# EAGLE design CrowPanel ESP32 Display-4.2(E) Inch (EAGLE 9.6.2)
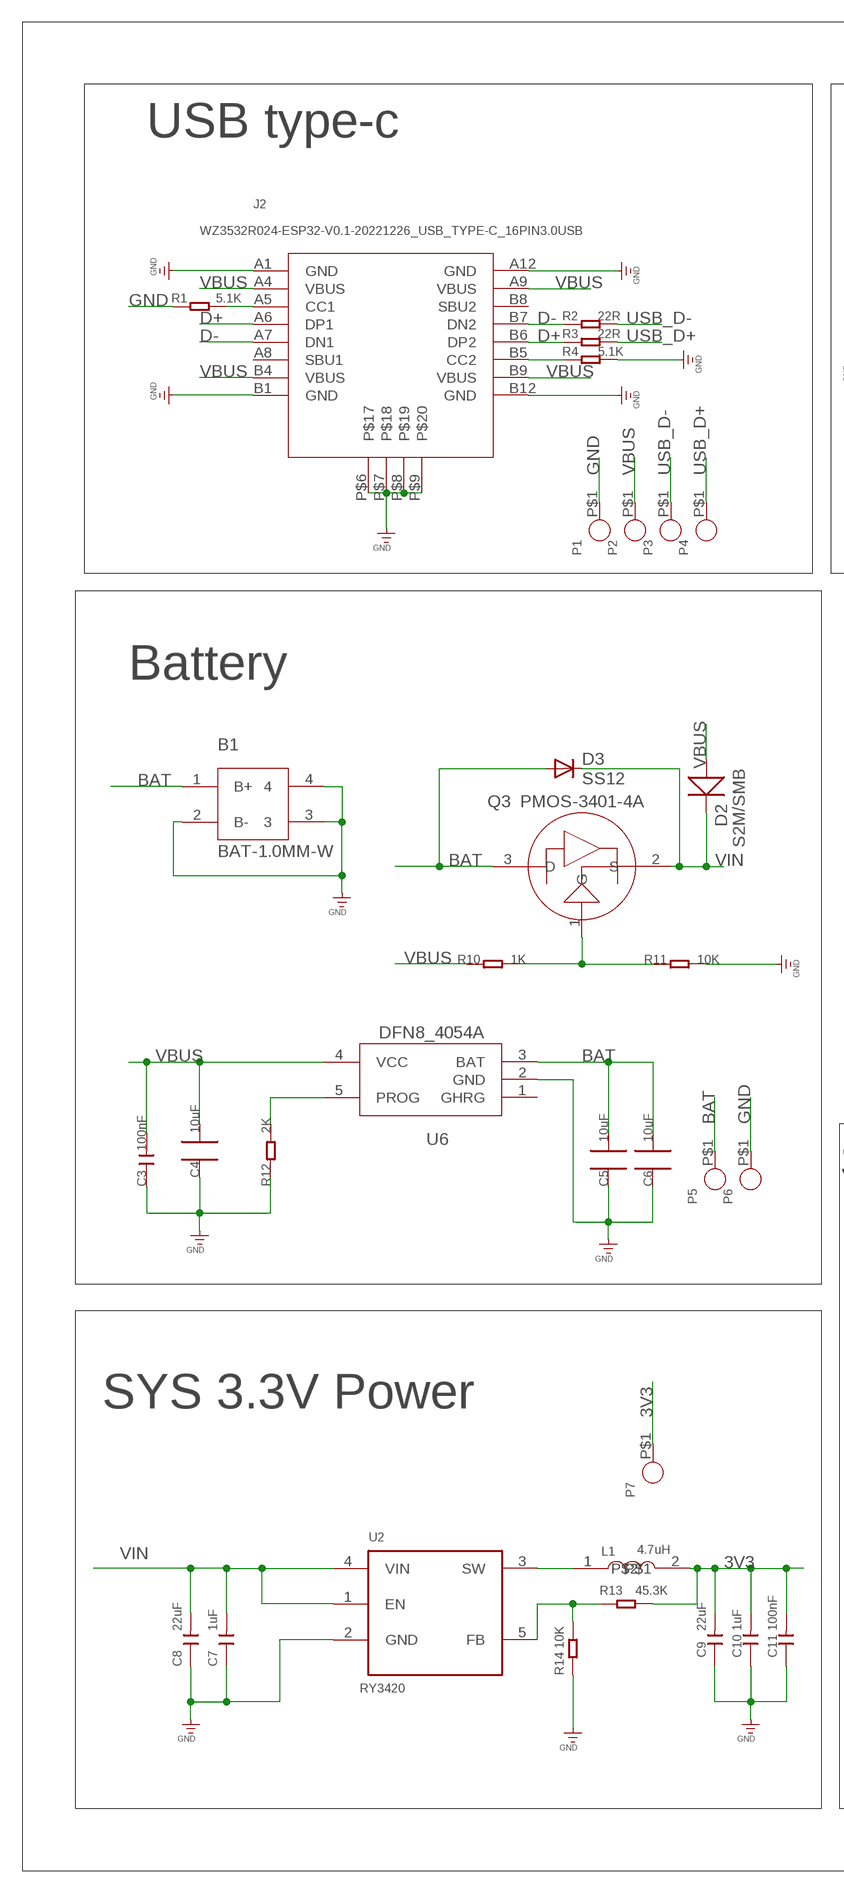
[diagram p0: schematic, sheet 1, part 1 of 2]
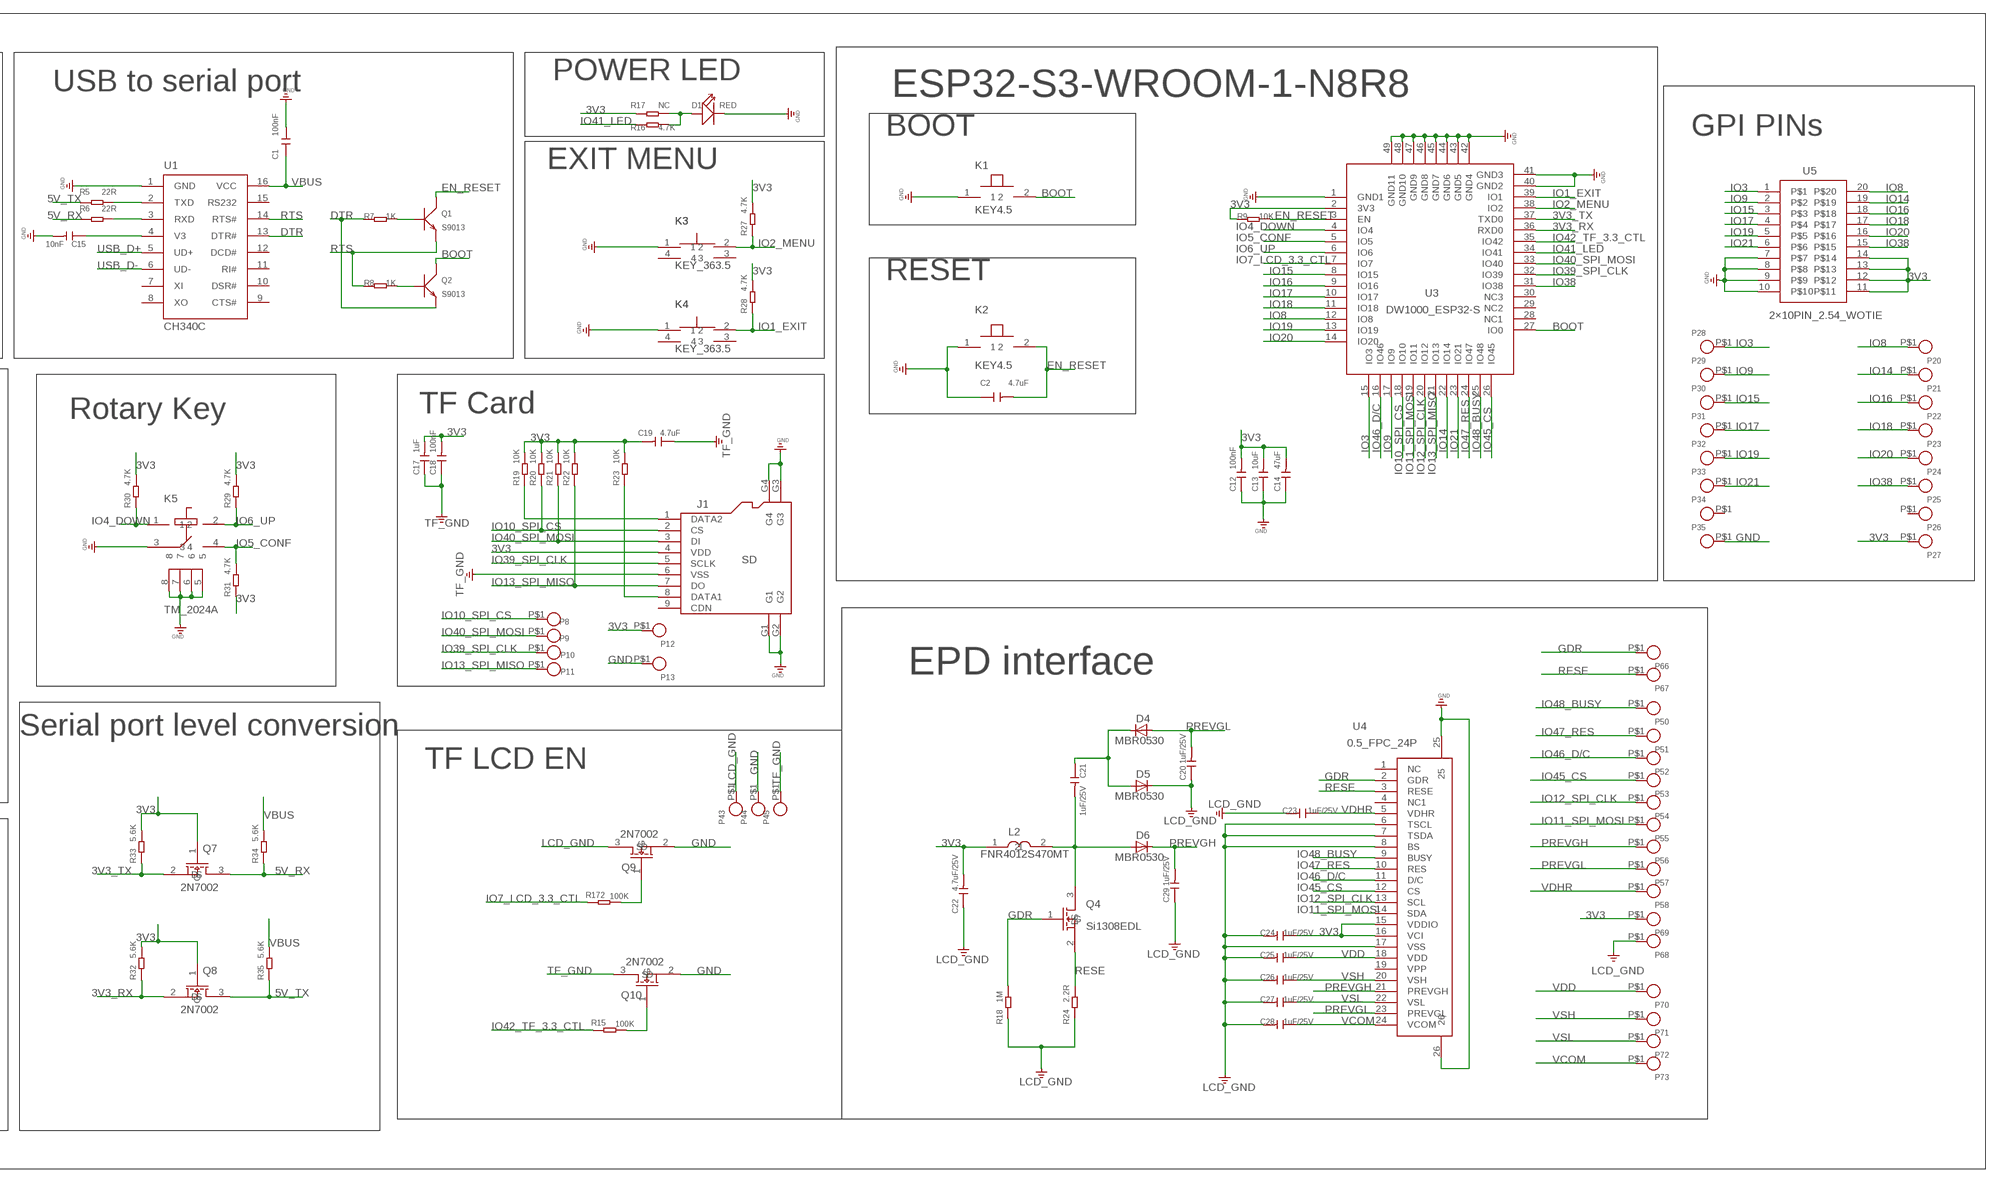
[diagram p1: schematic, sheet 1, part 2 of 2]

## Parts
B1  BAT-1.0MM-W  [SH1.0MM-W]
C1  100nF  C0603  [0603]
C2  4.7uF  A_XBJ_C0603  [A_XBJ_0603]
C3  100nF  A9G_DISCRETE_C-0603  [A9G_DISCRETE_C0603]
C4  10uF  CPT_SMD_C0805_S  [CPT_SMD_0805_S]
C5  10uF  CPT_SMD_C0805_S  [CPT_SMD_0805_S]
C6  10uF  CPT_SMD_C0805_S  [CPT_SMD_0805_S]
C7  1uF  A_XBJ_C0603  [A_XBJ_0603]
C8  22uF  A_XBJ_C0805  [A_XBJ_0805]
C9  22uF  A_XBJ_C0805  [A_XBJ_0805]
C10  1uF  A_XBJ_C0603  [A_XBJ_0603]
C11  100nF  A_XBJ_C0603  [A_XBJ_0603]
C12  100nF  A9G_DISCRETE_C-0603  [A9G_DISCRETE_C0603]
C13  10uF  A9G_DISCRETE_C-0603  [A9G_DISCRETE_C0603]
C14  47uF  A9G_DISCRETE_C-0805  [A9G_DISCRETE_C0805]
C15  10nF  A_XBJ_C0603  [A_XBJ_0603]
C17  1uF  A9G_DISCRETE_C-0603  [A9G_DISCRETE_C0603]
C18  100nF  A9G_DISCRETE_C-0603  [A9G_DISCRETE_C0603]
C19  4.7uF  A9G_DISCRETE_C-0603  [A9G_DISCRETE_C0603]
C20  1uF/25V  A9G_DISCRETE_C-0603  [A9G_DISCRETE_C0603]
C21  1uF/25V  A9G_DISCRETE_C-0603  [A9G_DISCRETE_C0603]
C22  4.7uF/25V  A9G_DISCRETE_C-0603  [A9G_DISCRETE_C0603]
C23  1uF/25V  A9G_DISCRETE_C-0603  [A9G_DISCRETE_C0603]
C24  1uF/25V  A9G_DISCRETE_C-0603  [A9G_DISCRETE_C0603]
C25  1uF/25V  A9G_DISCRETE_C-0603  [A9G_DISCRETE_C0603]
C26  1uF/25V  A9G_DISCRETE_C-0603  [A9G_DISCRETE_C0603]
C27  1uF/25V  A9G_DISCRETE_C-0603  [A9G_DISCRETE_C0603]
C28  1uF/25V  A9G_DISCRETE_C-0603  [A9G_DISCRETE_C0603]
C29  1uF/25V  A9G_DISCRETE_C-0603  [A9G_DISCRETE_C0603]
D1  RED  A_XBJ_DISCRETE_LED0603  [A_XBJ_DISCRETE_LED-0603]
D2  S2M/SMB  DO-214AB_214ABDO-214AB  [DO-214AB_214AB]
D3  SS12  DIODE_DIODE-DO-214AC  [DIODE_DO-214AC]
D4  MBR0530  DIODE_DIODE-SOD123  [DIODE_SOD123]
D5  MBR0530  DIODE_DIODE-SOD123  [DIODE_SOD123]
D6  MBR0530  DIODE_DIODE-SOD123  [DIODE_SOD123]
J1  SD  CONNECTOR_HOLDER-MICROSD-9P  [CONNECTOR_9P-SMD-W/-RING]
J2  WZ3532R024-ESP32-V0.1-20221226_USB_TYPE-C_16PIN3.0USB  [WZ3532R024-ESP32-V0.1-20221226_KEVIN_3.0TYPEC-SMD]
K1  KEY4.5  [KEY-4.5]
K2  KEY4.5  [KEY-4.5]
K3  KEY_363.5  [KEY_3*6*3.5]
K4  KEY_363.5  [KEY_3*6*3.5]
K5  TM_2024A  [TM_2024A]
L1  4.7uH  WZ2432R028-ESP32-V1.2-20231108_L-0530  [WZ2432R028-ESP32-V1.2-20231108_CD54_CD54]
L2  FNR4012S470MT  [FNR4012S470MT]
P1  CROWPI_POW_PADPAD-1.0MM  [CROWPI_POW_PAD-1.0MM]
P2  CROWPI_POW_PADPAD-1.0MM  [CROWPI_POW_PAD-1.0MM]
P3  CROWPI_POW_PADPAD-1.0MM  [CROWPI_POW_PAD-1.0MM]
P4  CROWPI_POW_PADPAD-1.0MM  [CROWPI_POW_PAD-1.0MM]
P5  CROWPI_POW_PADPAD-1.0MM  [CROWPI_POW_PAD-1.0MM]
P6  CROWPI_POW_PADPAD-1.0MM  [CROWPI_POW_PAD-1.0MM]
P7  CROWPI_POW_PADPAD-1.0MM  [CROWPI_POW_PAD-1.0MM]
P8  CROWPI_POW_PADPAD-1.0MM  [CROWPI_POW_PAD-1.0MM]
P9  CROWPI_POW_PADPAD-1.0MM  [CROWPI_POW_PAD-1.0MM]
P10  CROWPI_POW_PADPAD-1.0MM  [CROWPI_POW_PAD-1.0MM]
P11  CROWPI_POW_PADPAD-1.0MM  [CROWPI_POW_PAD-1.0MM]
P12  CROWPI_POW_PADPAD-1.0MM  [CROWPI_POW_PAD-1.0MM]
P13  CROWPI_POW_PADPAD-1.0MM  [CROWPI_POW_PAD-1.0MM]
P20  CROWPI_POW_PADPAD-1.0MM  [CROWPI_POW_PAD-1.0MM]
P21  CROWPI_POW_PADPAD-1.0MM  [CROWPI_POW_PAD-1.0MM]
P22  CROWPI_POW_PADPAD-1.0MM  [CROWPI_POW_PAD-1.0MM]
P23  CROWPI_POW_PADPAD-1.0MM  [CROWPI_POW_PAD-1.0MM]
P24  CROWPI_POW_PADPAD-1.0MM  [CROWPI_POW_PAD-1.0MM]
P25  CROWPI_POW_PADPAD-1.0MM  [CROWPI_POW_PAD-1.0MM]
P26  CROWPI_POW_PADPAD-1.0MM  [CROWPI_POW_PAD-1.0MM]
P27  CROWPI_POW_PADPAD-1.0MM  [CROWPI_POW_PAD-1.0MM]
P28  CROWPI_POW_PADPAD-1.0MM  [CROWPI_POW_PAD-1.0MM]
P29  CROWPI_POW_PADPAD-1.0MM  [CROWPI_POW_PAD-1.0MM]
P30  CROWPI_POW_PADPAD-1.0MM  [CROWPI_POW_PAD-1.0MM]
P31  CROWPI_POW_PADPAD-1.0MM  [CROWPI_POW_PAD-1.0MM]
P32  CROWPI_POW_PADPAD-1.0MM  [CROWPI_POW_PAD-1.0MM]
P33  CROWPI_POW_PADPAD-1.0MM  [CROWPI_POW_PAD-1.0MM]
P34  CROWPI_POW_PADPAD-1.0MM  [CROWPI_POW_PAD-1.0MM]
P35  CROWPI_POW_PADPAD-1.0MM  [CROWPI_POW_PAD-1.0MM]
P43  CROWPI_POW_PADPAD-1.0MM  [CROWPI_POW_PAD-1.0MM]
P44  CROWPI_POW_PADPAD-1.0MM  [CROWPI_POW_PAD-1.0MM]
P45  CROWPI_POW_PADPAD-1.0MM  [CROWPI_POW_PAD-1.0MM]
P50  CROWPI_POW_PADPAD-1.0MM  [CROWPI_POW_PAD-1.0MM]
P51  CROWPI_POW_PADPAD-1.0MM  [CROWPI_POW_PAD-1.0MM]
P52  CROWPI_POW_PADPAD-1.0MM  [CROWPI_POW_PAD-1.0MM]
P53  CROWPI_POW_PADPAD-1.0MM  [CROWPI_POW_PAD-1.0MM]
P54  CROWPI_POW_PADPAD-1.0MM  [CROWPI_POW_PAD-1.0MM]
P55  CROWPI_POW_PADPAD-1.0MM  [CROWPI_POW_PAD-1.0MM]
P56  CROWPI_POW_PADPAD-1.0MM  [CROWPI_POW_PAD-1.0MM]
P57  CROWPI_POW_PADPAD-1.0MM  [CROWPI_POW_PAD-1.0MM]
P58  CROWPI_POW_PADPAD-1.0MM  [CROWPI_POW_PAD-1.0MM]
P66  CROWPI_POW_PADPAD-1.0MM  [CROWPI_POW_PAD-1.0MM]
P67  CROWPI_POW_PADPAD-1.0MM  [CROWPI_POW_PAD-1.0MM]
P68  CROWPI_POW_PADPAD-1.0MM  [CROWPI_POW_PAD-1.0MM]
P69  CROWPI_POW_PADPAD-1.0MM  [CROWPI_POW_PAD-1.0MM]
P70  CROWPI_POW_PADPAD-1.0MM  [CROWPI_POW_PAD-1.0MM]
P71  CROWPI_POW_PADPAD-1.0MM  [CROWPI_POW_PAD-1.0MM]
P72  CROWPI_POW_PADPAD-1.0MM  [CROWPI_POW_PAD-1.0MM]
P73  CROWPI_POW_PADPAD-1.0MM  [CROWPI_POW_PAD-1.0MM]
Q1  S9013  DISCRETE_TRANSISTOR-NPN-SOT23  [DISCRETE_SOT23$1]
Q2  S9013  DISCRETE_TRANSISTOR-NPN-SOT23  [DISCRETE_SOT23$1]
Q3  PMOS-3401-4A  DFN8_P-MOS-SOT23  [DFN8_SOT-23]
Q4  Si1308EDL  HXY2102EI  [SOT-323_W]
Q7  2N7002  NMOS_W  [SOT23-3_W]
Q8  2N7002  NMOS_W  [SOT23-3_W]
Q9  2N7002  NMOS_W  [SOT23-3_W]
Q10  2N7002  NMOS_W  [SOT23-3_W]
R1  5.1K  R0603  [R0603]
R2  22R  R0603  [R0603]
R3  22R  R0603  [R0603]
R4  5.1K  R0603  [R0603]
R5  22R  R0603  [R0603]
R6  22R  R0603  [R0603]
R7  1K  A9G_DISCRETE_R-0603  [A9G_DISCRETE_R0603]
R8  1K  A9G_DISCRETE_R-0603  [A9G_DISCRETE_R0603]
R9  10K  A9G_DISCRETE_R-0603  [A9G_DISCRETE_R0603]
R10  1K  A9G_DISCRETE_R-0603  [A9G_DISCRETE_R0603]
R11  10K  A9G_DISCRETE_R-0603  [A9G_DISCRETE_R0603]
R12  2K  A9G_DISCRETE_R-0603  [A9G_DISCRETE_R0603]
R13  45.3K  A9G_DISCRETE_R-0603  [A9G_DISCRETE_R0603]
R14  10K  A9G_DISCRETE_R-0603  [A9G_DISCRETE_R0603]
R15  100K  R-0603  [R0603]
R16  4.7K  A9G_DISCRETE_R-0603  [A9G_DISCRETE_R0603]
R17  NC  A9G_DISCRETE_R-0603  [A9G_DISCRETE_R0603]
R18  1M  A9G_DISCRETE_R-0603  [A9G_DISCRETE_R0603]
R19  10K  A9G_DISCRETE_R-0603  [A9G_DISCRETE_R0603]
R20  10K  A9G_DISCRETE_R-0603  [A9G_DISCRETE_R0603]
R21  10K  A9G_DISCRETE_R-0603  [A9G_DISCRETE_R0603]
R22  10K  A9G_DISCRETE_R-0603  [A9G_DISCRETE_R0603]
R23  10K  A9G_DISCRETE_R-0603  [A9G_DISCRETE_R0603]
R24  2.2R  A9G_DISCRETE_R-0603  [A9G_DISCRETE_R0603]
R27  4.7K  A9G_DISCRETE_R-0603  [A9G_DISCRETE_R0603]
R28  4.7K  A9G_DISCRETE_R-0603  [A9G_DISCRETE_R0603]
R29  4.7K  A9G_DISCRETE_R-0603  [A9G_DISCRETE_R0603]
R30  4.7K  A9G_DISCRETE_R-0603  [A9G_DISCRETE_R0603]
R31  4.7K  A9G_DISCRETE_R-0603  [A9G_DISCRETE_R0603]
R32  5.6K  DISCRETE_R-0603  [DISCRETE_R0603]
R33  5.6K  DISCRETE_R-0603  [DISCRETE_R0603]
R34  5.6K  DISCRETE_R-0603  [DISCRETE_R0603]
R35  5.6K  DISCRETE_R-0603  [DISCRETE_R0603]
R172  100K  R-0603  [R0603]
U1  CH340C  A_XBJ_CH340G  [A_XBJ_SOP-16]
U2  RY3420  CROWBOT_-V1.0-20220525_A_XBJ_HM3420B  [CROWBOT_-V1.0-20220525_A_XBJ_SOT23-5]
U3  DW1000_ESP32-S  [DW1000_ESP32-S3]
U4  0.5_FPC_24P  [0.5_FPC_24P]
U5  2×10PIN_2.54_WOTIE  [2*10PIN_2.54_WOTIE]
U6  DFN8_4054A  [DFN8_SOP23-5]

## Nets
3V3: C9.2 C10.2 C11.2 C12.2 C13.2 C14.2 C17.2 C18.2 C19.2 C22.2 C24.1 J1.4(VDD) L1.2 L2.1 P7.P$1 P12.P$1 P27.P$1 P69.P$1 Q7.1(G) Q8.1(G) R9.1 R13.2 R17.1 R19.2 R20.2 R21.2 R22.2 R23.2 R27.2 R28.2 R29.2 R30.2 R31.1 R32.2 R33.2 U3.2(3V3) U4.15(VDDIO) U4.16(VCI) U5.11 U5.12 U5.13 U5.14
3V3_RX: Q8.2(S) R32.1 U3.36(RXD0)
3V3_TX: Q7.2(S) R33.1 U3.37(TXD0)
5V_RX: Q7.3(D) R6.1 R34.1
5V_TX: Q8.3(D) R5.1 R35.1
BAT: B1.1(B+) C5.2 C6.2 D3.A P5.P$1 Q3.3(D) U6.3(BAT)
BOOT: K1.2 Q2.3(C) U3.27(IO0)
D+: J2.A6(DP1) J2.B6(DP2) R3.1
D-: J2.A7(DN1) J2.B7(DN2) R2.1
DTR: Q2.2(E) R7.1 U1.13(DTR#)
EN_RESET: C2.2 K2.2 Q1.3(C) R9.2 U3.3(EN)
GDR: P66.P$1 Q4.1(G) R18.2 U4.2(GDR)
GND: B1.2(B-) B1.3 B1.4 C1.2 C2.1 C3.1 C4.1 C5.1 C6.1 C7.1 C8.1 C9.1 C10.1 C11.1 C12.1 C13.1 C14.1 C15.2 D1.- J1.G1 J1.G2 J1.G3 J1.G4 J2.A1(GND) J2.A12(GND) J2.B1(GND) J2.B12(GND) J2.P$6 J2.P$7 J2.P$8 J2.P$9 K1.1 K2.1 K3.1 K4.1 K5.3 K5.5 K5.6 K5.7 K5.8 P1.P$1 P6.P$1 P13.P$1 P35.P$1 P44.P$1 Q9.2(S) Q10.2(S) R1.1 R4.2 R11.2 R12.1 R14.1 U1.1(GND) U2.2(GND) U3.1(GND1) U3.40(GND2) U3.41(GND3) U3.42(GND4) U3.43(GND5) U3.44(GND6) U3.45(GND7) U3.46(GND8) U3.47(GND9) U3.48(GND10) U3.49(GND11) U4.25 U4.26 U5.7 U5.8 U5.9 U5.10 U6.2(GND)
IO1_EXIT: K4.2 R28.1 U3.39(IO1)
IO2_MENU: K3.2 R27.1 U3.38(IO2)
IO3: P28.P$1 U3.15(IO3) U5.1
IO4_DOWN: K5.1 R30.1 U3.4(IO4)
IO5_CONF: K5.4 R31.2 U3.5(IO5)
IO6_UP: K5.2 R29.1 U3.6(IO6)
IO7_LCD_3.3_CTL: R172.1 U3.7(IO7)
IO8: P20.P$1 U3.12(IO8) U5.20
IO9: P29.P$1 U3.17(IO9) U5.2
IO10_SPI_CS: J1.2(CS) P8.P$1 R20.1 U3.18(IO10)
IO11_SPI_MOSI: P55.P$1 U3.19(IO11) U4.14(SDA)
IO12_SPI_CLK: P54.P$1 U3.20(IO12) U4.13(SCL)
IO13_SPI_MISO: J1.7(DO) P11.P$1 R22.1 U3.21(IO13)
IO14: P21.P$1 U3.22(IO14) U5.19
IO15: P30.P$1 U3.8(IO15) U5.3
IO16: P22.P$1 U3.9(IO16) U5.18
IO17: P31.P$1 U3.10(IO17) U5.4
IO18: P23.P$1 U3.11(IO18) U5.17
IO19: P32.P$1 U3.13(IO19) U5.5
IO20: P24.P$1 U3.14(IO20) U5.16
IO21: P33.P$1 U3.23(IO21) U5.6
IO38: P25.P$1 U3.31(IO38) U5.15
IO39_SPI_CLK: J1.5(SCLK) P10.P$1 U3.32(IO39)
IO40_SPI_MOSI: J1.3(DI) P9.P$1 R21.1 U3.33(IO40)
IO41_LED: R16.1 U3.34(IO41)
IO42_TF_3.3_CTL: R15.1 U3.35(IO42)
IO45_CS: P53.P$1 U3.26(IO45) U4.12(CS)
IO46_D/C: P52.P$1 U3.16(IO46) U4.11(D/C)
IO47_RES: P51.P$1 U3.24(IO47) U4.10(RES)
IO48_BUSY: P50.P$1 U3.25(IO48) U4.9(BUSY)
LCD_GND: C20.1 C22.1 C23.2 C24.2 C25.2 C26.2 C27.2 C28.2 C29.1 D5.C P43.P$1 P68.P$1 Q9.3(D) R18.1 R24.1 U4.6(TSCL) U4.7(TSDA) U4.8(BS) U4.17(VSS) ; supply symbol labelled GND
N$1: Q1.1(B) R7.2
N$2: R5.2 U1.2(TXD)
N$3: R6.2 U1.3(RXD)
N$4: Q2.1(B) R8.2
N$5: J2.A5(CC1) R1.2
N$6: Q3.1(G) R10.2 R11.1
N$7: Q9.1(G) R172.2
N$8: Q10.1(G) R15.2
N$9: R13.1 R14.2 U2.5(FB)
N$10: J1.1(DATA2) R19.1
N$11: L1.1 U2.3(SW)
N$12: J2.B5(CC2) R4.1
N$13: C15.1 U1.4(V3)
N$16: R12.2 U6.5(PROG)
N$20: J1.8(DATA1) R23.1
N$25: D1.+ R16.2 R17.2
N$55: C21.1 D4.C D5.A
N$56: C21.2 D6.A L2.2 Q4.3(D)
PREVGH: C29.2 D6.C P56.P$1 U4.21(PREVGH)
PREVGL: C20.2 D4.A P57.P$1 U4.23(PREVGL)
RESE: P67.P$1 Q4.2(S) R24.2 U4.3(RESE)
RTS: Q1.2(E) R8.1 U1.14(RTS#)
TF_GND: C17.1 C18.1 C19.1 J1.6(VSS) P45.P$1 Q10.3(D) ; supply symbol labelled GND
USB_D+: P4.P$1 R3.2 U1.5(UD+)
USB_D-: P3.P$1 R2.2 U1.6(UD-)
VBUS: C1.1 C3.2 C4.2 D2.1(+) J2.A4(VBUS) J2.A9(VBUS) J2.B4(VBUS) J2.B9(VBUS) P2.P$1 R10.1 R34.2 R35.2 U1.16(VCC) U6.4(VCC)
VCOM: C28.1 P73.P$1 U4.24(VCOM)
VDD: C25.1 P70.P$1 U4.18(VDD)
VDHR: C23.1 P58.P$1 U4.5(VDHR)
VIN: C7.2 C8.2 D2.2(-) D3.C Q3.2(S) U2.1(EN) U2.4(VIN)
VSH: C26.1 P71.P$1 U4.20(VSH)
VSL: C27.1 P72.P$1 U4.22(VSL)
Unconnected: J1.9(CDN) J2.A8(SBU1) J2.B8(SBU2) K3.3 K3.4 K4.3 K4.4 P26.P$1 P34.P$1 U1.7(XI) U1.8(XO) U1.9(CTS#) U1.10(DSR#) U1.11(RI#) U1.12(DCD#) U1.15(RS232) U3.28(NC1) U3.29(NC2) U3.30(NC3) U4.1(NC) U4.4(NC1) U4.19(VPP) U6.1(GHRG)

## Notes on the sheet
- USB type-c | POWER LED
- USB to serial port | ESP32-S3-WROOM-1-N8R8
- BOOT | GPI PINs
- EXIT MENU
- RESET
- Rotary Key | TF Card
- Battery
- EPD interface
- Serial port level conversion
- TF LCD EN
- SYS 3.3V Power

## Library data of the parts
B1 = WGH:BAT-1.0MM-W
C1 = WGH:C0603
C2 C7 C10 C11 C15 = CrowPanel ESP32 Display-4.3-inch-V2.1-20240314:A_XBJ_C0603
C3 C12-C14 C17-C29 = CrowPanel ESP32 Display-4.3-inch-V2.1-20240314:A9G_DISCRETE_C*: Ceramic Capacitors
C4-C6 = CrowPanel ESP32 Display-4.3-inch-V2.1-20240314:CPT_SMD_C0805
C8 C9 = CrowPanel ESP32 Display-4.3-inch-V2.1-20240314:A_XBJ_C0805
D1 = CrowPanel ESP32 Display-4.3-inch-V2.1-20240314:A_XBJ_DISCRETE_LED*
D2 = CrowPanel ESP32 Display-4.3-inch-V2.1-20240314:DO-214AB_214AB: 214AB
D3-D6 = CrowPanel ESP32 Display-4.3-inch-V2.1-20240314:DIODE_DIODE-: DIODE
J1 = CrowPanel ESP32 Display-4.3-inch-V2.1-20240314:CONNECTOR_HOLDER-MICROSD-9P
J2 = CrowPanel ESP32 Display-4.3-inch-V2.1-20240314:WZ3532R024-ESP32-V0.1-20221226_USB_TYPE-C_16PIN
K1 K2 = WGH:KEY4.5
K3 K4 = WGH:KEY_3*6*3.5
K5 = WGH:TM_2024A
L1 = CrowPanel ESP32 Display-4.3-inch-V2.1-20240314:WZ2432R028-ESP32-V1.2-20231108_L-0530
L2 = WGH:FNR4012S470MT
P1-P13 P20-P35 P43-P45 P50-P58 P66-P73 = ESP32 Terminal - 3.5 Inch_2.0:CROWPI_POW_PAD*
Q1 Q2 = CrowPanel ESP32 Display-4.3-inch-V2.1-20240314:DISCRETE_TRANSISTOR-NPN*: NPN audion
Q3 = CrowPanel ESP32 Display-4.3-inch-V2.1-20240314:DFN8_P-MOS-SOT23
Q4 = WGH:HXY2102EI
Q7-Q10 = WGH:NMOS_W
R1-R6 = WGH:R0603
R7-R14 R16-R24 R27-R31 = CrowPanel ESP32 Display-4.3-inch-V2.1-20240314:A9G_DISCRETE_R*
R15 R172 = discrete:R*
R32-R35 = CrowPanel ESP32 Display-4.3-inch-V2.1-20240314:DISCRETE_R*
U1 = CrowPanel ESP32 Display-4.3-inch-V2.1-20240314:A_XBJ_CH340G
U2 = CrowPanel ESP32 Display-4.3-inch-V2.1-20240314:CROWBOT_-V1.0-20220525_A_XBJ_HM3420B
U3 = CrowPanel ESP32 Display-4.3-inch-V2.1-20240314:DW1000_ESP32-S
U4 = ESP32 Terminal - 3.5 Inch_2.0:0.5_FPC_24P
U5 = WGH:2×10PIN_2.54_WOTIE
U6 = CrowPanel ESP32 Display-4.3-inch-V2.1-20240314:DFN8_4054A

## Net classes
0 default: width 0.254 mm, drill 0.305 mm, clearance 0.152 mm

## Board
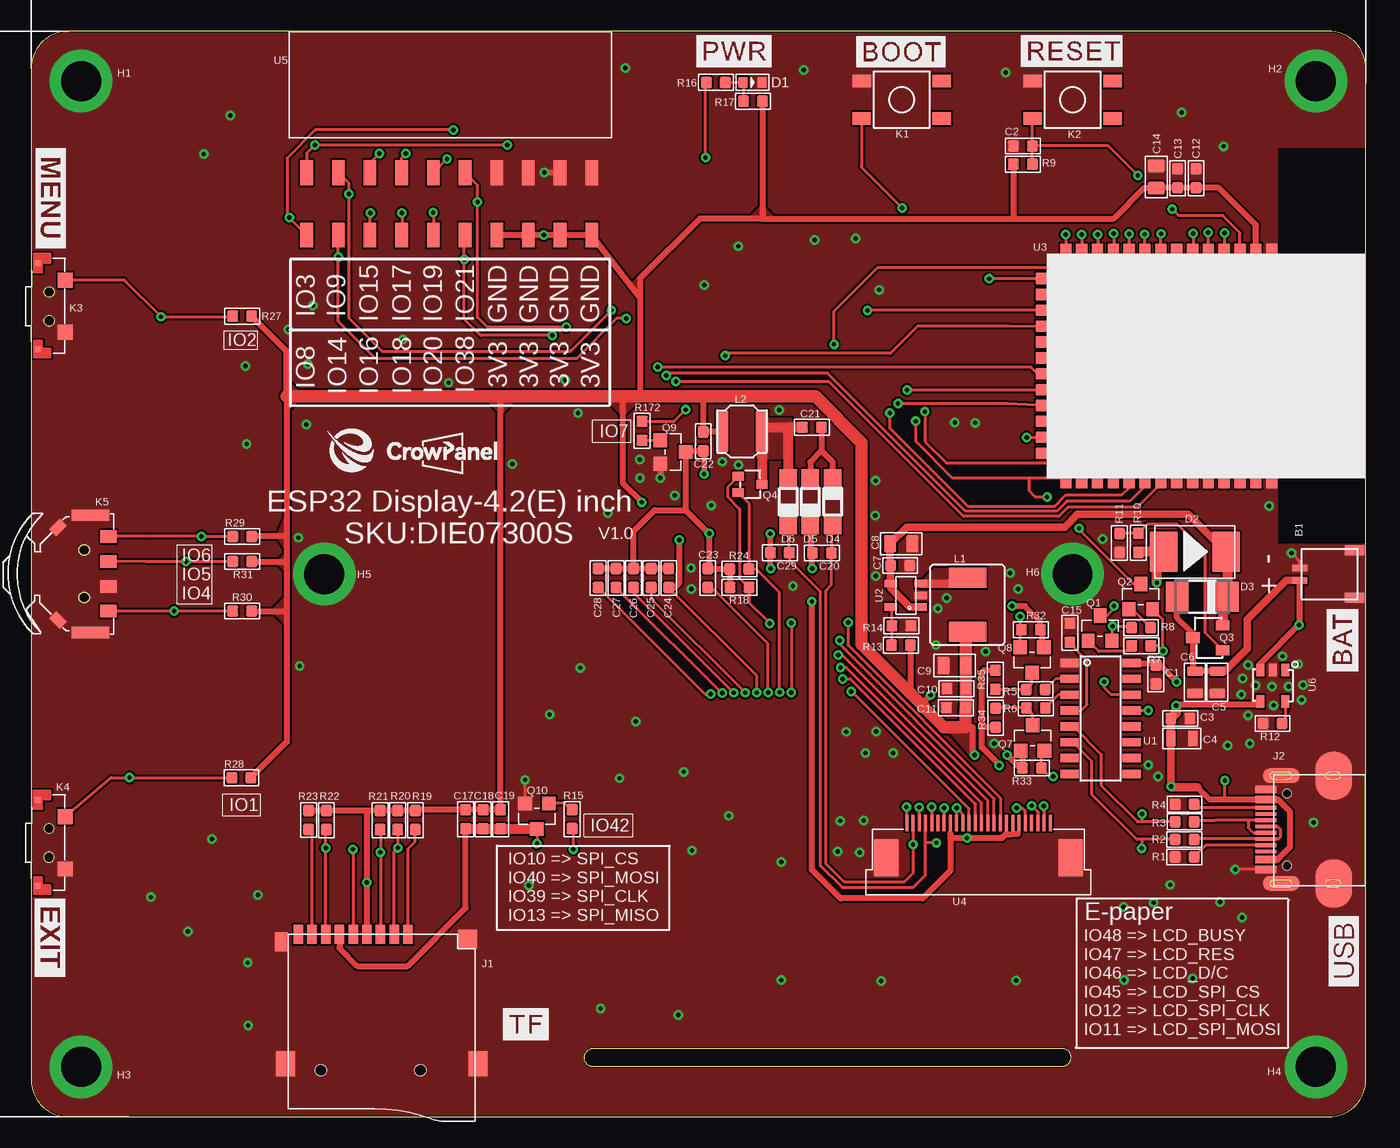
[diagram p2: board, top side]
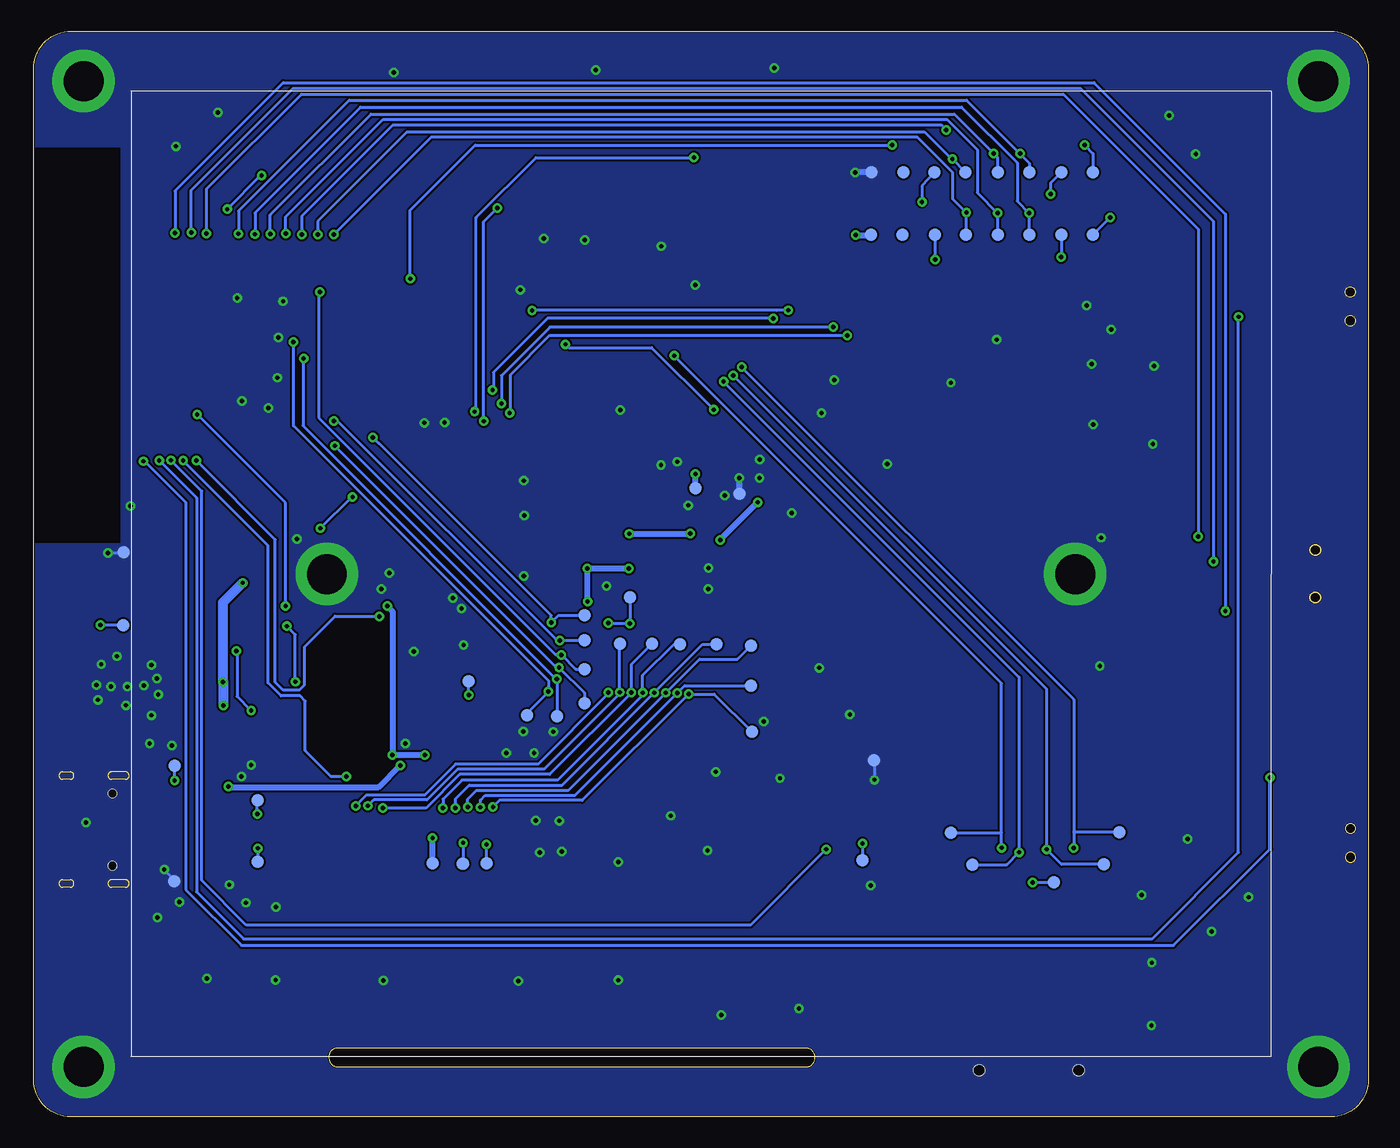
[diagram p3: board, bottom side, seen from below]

Size 107 x 87 mm. Coordinates in mm from the lower left corner, seen from the top.
Outline: 0,84.01 0,2.98 arc90 2.98,0 104.03,0 arc90 107,2.97 107,84.01 arc90 104.01,87 2.99,87 arc90 0,84.01
Outline: 83.34,4.81 83.34,4.75 arc-90 82.59,3.99 45.1,3.99 arc-90 44.35,4.71 44.35,4.76 arc-90 45.1,5.5 82.61,5.5 arc-90 83.34,4.81
Copper layers (1*16): Top 0.035mm / dielectric 1.5mm / Bottom 0.035mm
Design rules "default *": minimum track width 6mil, minimum drill 0.35mm, track to track 6mil, track to pad 6mil, pad to pad 6mil, via to via 6mil, smd to smd 6mil, copper to edge 2mil, drill to drill 6mil, minimum pad ring 10mil, minimum via ring 8mil, stop-mask expansion 4mil, vias tented up to drill 100mil, thermal gap 0mil

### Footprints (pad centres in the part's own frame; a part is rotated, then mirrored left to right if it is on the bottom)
SH1.0MM-W = smd 0.5 x 1.2: 1 -0.5,2.4; 2 0.5,2.4 | smd 0.8 x 1.6: 3 -1.9,-2; 4 1.9,-2
0603 = smd 0.889 x 0.889: 1 -0.762,0; 2 0.762,0
A_XBJ_0603 = smd 0.889 x 0.889: 1 -0.762,0; 2 0.762,0
A9G_DISCRETE_C0603 = smd 0.889 x 0.889: 1 -0.762,0; 2 0.762,0
CPT_SMD_0805_S = smd 0.762 x 1.27: 1 -0.889,0; 2 0.889,0
A_XBJ_0805 = smd 1.016 x 1.397: 1 -0.889,0; 2 0.889,0
A9G_DISCRETE_C0805 = smd 1.016 x 1.397: 1 -0.889,0; 2 0.889,0
A_XBJ_DISCRETE_LED-0603 = smd 0.762 x 0.889: + -0.762,0; - 0.762,0
DO-214AB_214AB = smd 2.2 x 3.2: 1 -2.5,0; 2 2.5,0
DIODE_DO-214AC = smd 1.8 x 2.4: A 2.025,0; C -2.025,0
DIODE_SOD123 = smd 1.4 x 1.4: A 1.9,0; C -1.9,0
CONNECTOR_9P-SMD-W/-RING = smd 1.524 x 0.762: 1 0,4.4; 2 0,3.3; 3 0,2.2; 4 0,1.1; 5 0,0; 6 0,-1.1; 7 0,-2.2; 8 0,-3.3; 9 0,-4.4 | smd 1.524 x 1.016: G1 0.6,-5.746 | smd 2.032 x 1.524: G2 10.373,-5.4; G3 10.373,10 | smd 1.524 x 1.524: G4 0.392,9.181 | hole 0.889: 10.9,-2.6; 10.9,5.4
WZ3532R024-ESP32-V0.1-20221226_KEVIN_3.0TYPEC-SMD = smd 0.3 x 1.7: A1 -3.35,0.5; A4 -2.55,0.5; A5 -1.25,0.5; A6 -0.25,0.5; A7 0.25,0.5; A8 1.25,0.5; A9 2.55,0.5; A12 3.35,0.5; B1 3.05,0.5; B4 2.25,0.5; B5 1.75,0.5; B6 0.75,0.5; B7 -0.75,0.5; B8 -1.75,0.5; B9 -2.25,0.5; B12 -3.05,0.5 | smd 1.143 x 2.921: P$6 -4.318,-0.762; P$7 4.318,-0.762 | smd 3.81 x 2.921: P$8 -4.318,-4.953; P$9 4.318,-4.953 | hole 0.68: -2.89,-1.22; 2.89,-1.22
KEY-4.5 = smd 1.5 x 1: 1 -3.2,1.5; 2 -3.2,-1.5; 3 3.2,-1.5; 4 3.2,1.5
KEY_3*6*3.5 = smd 1.2 x 1.2: 1 -2.1,-2.6; 2 2.1,-2.6 | smd 0.5 x 0.5: 3 3.45,-0.4; 4 -3.45,-0.4
TM_2024A = smd 1 x 1.3: 1 -3,0.65; 2 3,0.65; 3 -1,0.65; 4 1,0.65 | smd 0.9 x 3: 5 -4.7,2.1; 6 4.7,2.1 | smd 1.2 x 0.8 rotated 45: 7 -3.7,4.7 | smd 1.2 x 0.8 rotated 135: 8 3.7,4.7
WZ2432R028-ESP32-V1.2-20231108_CD54_CD54 = smd 3 x 1.6: 1 0,2.159; 2 0,-2.159
FNR4012S470MT = smd 0.95 x 3.3: 1 -1.6,0; 2 1.6,0
CROWPI_POW_PAD-1.0MM = smd 1 x 1: P$1 0,0
DISCRETE_SOT23$1 = smd 1.016 x 1.143: 1 -0.95,-1.016; 2 0.95,-1.016; 3 0,1.016
DFN8_SOT-23 = smd 1.1 x 0.8: 1 1.2,-1; 2 1.2,1 | smd 1.1 x 0.9: 3 -1.2,0
SOT-323_W = smd 0.7 x 0.9: 1 -0.65,-0.95; 2 0.65,-0.95; 3 0,0.95
SOT23-3_W = smd 1.1 x 1.1: 1 -0.95,-1.016; 2 0.95,-1.016; 3 0,1.016
R0603 = smd 0.889 x 0.889: 1 -0.762,0; 2 0.762,0
A9G_DISCRETE_R0603 = smd 0.889 x 0.889: 1 -0.762,0; 2 0.762,0
DISCRETE_R0603 = smd 0.889 x 0.889: 1 -0.762,0; 2 0.762,0
A_XBJ_SOP-16 = smd 0.66 x 1.5: 1 -4.445,-2.475; 2 -3.175,-2.475; 3 -1.905,-2.475; 4 -0.635,-2.475; 5 0.635,-2.475; 6 1.905,-2.475; 7 3.175,-2.475; 8 4.445,-2.475; 9 4.445,2.475; 10 3.175,2.475; 11 1.905,2.475; 12 0.635,2.475; 13 -0.635,2.475; 14 -1.905,2.475; 15 -3.175,2.475; 16 -4.445,2.475
CROWBOT_-V1.0-20220525_A_XBJ_SOT23-5 = smd 0.6 x 1: 1 -0.95,-1.2; 2 0,-1.2; 3 0.95,-1.2; 4 0.95,1.2; 5 -0.95,1.2
DW1000_ESP32-S3 = smd 1.6 x 0.9: 1 0,18.01; 2 0,16.74; 3 0,15.47; 4 0,14.2; 5 0,12.93; 6 0,11.66; 7 0,10.39; 8 0,9.12; 9 0,7.85; 10 0,6.58; 11 0,5.31; 12 0,4.04; 13 0,2.77; 14 0,1.5; 27 18,1.5; 28 18,2.77; 29 18,4.04; 30 18,5.31; 31 18,6.58; 32 18,7.85; 33 18,9.12; 34 18,10.39; 35 18,11.66; 36 18,12.93; 37 18,14.2; 38 18,15.47; 39 18,16.74; 40 18,18.01 | smd 0.9 x 1.8: 15 2,0; 16 3.28,0; 17 4.55,0; 18 5.82,0; 19 7.09,0; 20 8.36,0; 21 9.63,0; 22 10.9,0; 23 12.17,0; 24 13.44,0; 25 14.71,0; 26 16,0 | smd 1 x 1: 41 7.64,11.16; 42 9.14,11.16; 43 6.14,11.16; 44 6.14,14.16; 45 7.64,12.66; 46 9.14,12.66; 47 7.64,14.16; 48 9.14,14.16; 49 6.14,12.66
0.5_FPC_24P = smd 1.3 x 0.3: 1 -2.54,5.75; 2 -2.54,5.25; 3 -2.54,4.75; 4 -2.54,4.25; 5 -2.54,3.75; 6 -2.54,3.25; 7 -2.54,2.75; 8 -2.54,2.25; 9 -2.54,1.75; 10 -2.54,1.25; 11 -2.54,0.75; 12 -2.54,0.25; 13 -2.54,-0.25; 14 -2.54,-0.75; 15 -2.54,-1.25; 16 -2.54,-1.75; 17 -2.54,-2.25; 18 -2.54,-2.75; 19 -2.54,-3.25; 20 -2.54,-3.75; 21 -2.54,-4.25; 22 -2.54,-4.75; 23 -2.54,-5.25; 24 -2.54,-5.75 | smd 3 x 2: 25 0.27,-7.4; 26 0.27,7.4
2*10PIN_2.54_WOTIE = smd 1.02 x 2: 1 1.4,-7; 2 3.94,-7; 3 6.48,-7; 4 9.02,-7; 5 11.56,-7; 6 14.1,-7; 7 16.64,-7; 8 19.18,-7; 9 21.72,-7; 10 24.26,-7; 11 24.26,-12; 12 21.72,-12; 13 19.18,-12; 14 16.64,-12; 15 14.1,-12; 16 11.56,-12; 17 9.02,-12; 18 6.48,-12; 19 3.94,-12; 20 1.4,-12
DFN8_SOP23-5 = smd 1 x 0.635: 1 -1.27,1; 2 -1.27,0; 3 -1.27,-1; 4 1.27,-1; 5 1.27,1

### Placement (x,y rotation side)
B1  104.09,43.48 90 top
C1  90.17,35.44 270 top
C2  79.5,77.8 0 top
C3  92.13,31.91 180 top
C4  92.24,30.31 180 top
C5  95.09,34.82 90 top
C6  93.29,34.82 90 top
C7  69.66,44.17 180 top
C8  69.75,45.92 180 top
C9  74.04,36.16 0 top
C10  74.17,34.31 0 top
C11  74.14,32.77 0 top
C12  93.39,75.21 270 top
C13  91.91,75.21 270 top
C14  90.19,75.31 270 top
C15  83.27,38.78 90 top
C17  34.83,23.84 90 top
C18  36.23,23.84 90 top
C19  37.63,23.84 90 top
C20  63.39,45.18 0 top
C21  62.59,55.26 180 top
C22  53.88,54.12 90 top
C23  54.24,43.17 90 top
C24  51.11,43.17 90 top
C25  49.7,43.17 90 top
C26  48.29,43.17 90 top
C27  46.88,43.17 90 top
C28  45.45,43.17 90 top
C29  60.02,45.19 0 top
D1  57.83,82.89 0 top
D2  93.28,45.26 0 top
D3  93.88,41.67 180 top
D4  64.27,49.29 270 top
D5  62.46,49.28 90 top
D6  60.7,49.28 90 top
J1  25.81,14.62 270 top
J2  99.47,23.01 90 top
K1  69.79,81.51 0 top
K2  83.49,81.51 0 top
K3  KEY_36*3.5  [KEY_3*6*3.5]  0.14,64.95 90 top
K4  KEY_36*3.5  [KEY_3*6*3.5]  0.13,21.95 90 top
K5  6.85,43.51 90 top
L1  75.06,41.02 0 top
L2  56.98,54.93 0 top
P1  95.72,18.87 0 bottom
P2  95.7,28.12 0 bottom
P3  89.04,20.44 0 bottom
P4  89.05,25.35 0 bottom
P5  99.8,39.4 0 bottom
P6  99.79,45.22 0 bottom
P7  72.14,34.89 0 bottom
P8  33.45,22.76 0 bottom
P9  31.73,20.21 0 bottom
P10  21.19,20.23 0 bottom
P11  19.95,22.78 0 bottom
P12  25.19,18.78 0 bottom
P13  39.62,28.56 0 bottom
P20  22.08,70.69 0 bottom
P21  24.61,70.69 0 bottom
P22  27.17,70.69 0 bottom
P23  29.69,70.69 0 bottom
P24  32.26,70.69 0 bottom
P25  34.75,70.69 0 bottom
P26  37.34,70.69 0 bottom
P27  39.86,70.69 0 bottom
P28  22.07,75.68 0 bottom
P29  24.62,75.68 0 bottom
P30  27.15,75.68 0 bottom
P31  29.71,75.68 0 bottom
P32  32.28,75.68 0 bottom
P33  34.79,75.68 0 bottom
P34  37.26,75.68 0 bottom
P35  39.85,75.68 0 bottom
P43  53.92,50.36 0 bottom
P44  50.43,49.94 0 bottom
P45  40.55,20.54 0 bottom
P50  62.85,40.18 0 bottom
P51  62.85,38.17 0 bottom
P52  62.84,35.86 0 bottom
P53  62.85,33.15 0 bottom
P54  65.05,32.09 0 bottom
P55  67.46,32.16 0 bottom
P56  72.59,20.29 0 bottom
P57  70.69,20.32 0 bottom
P58  57.42,37.91 0 bottom
P66  59.2,41.63 0 bottom
P67  59.97,37.92 0 bottom
P68  75.02,20.3 0 bottom
P69  55.16,37.85 0 bottom
P70  52.25,37.85 0 bottom
P71  49.5,37.76 0 bottom
P72  49.48,34.55 0 bottom
P73  49.42,30.85 0 bottom
Q1  85.69,39.16 0 top
Q2  88.96,41.68 0 top
Q3  94.32,38.39 0 top
Q4  57.63,50.67 270 top
Q7  80.28,30.35 0 top
Q8  80.24,36.6 180 top
Q9  51.45,53.27 270 top
Q10  40.54,24.08 180 top
R1  92.46,20.81 0 top
R2  92.46,22.22 180 top
R3  92.47,23.63 180 top
R4  92.47,25.04 180 top
R5  80.52,34.23 0 top
R6  80.54,32.76 0 top
R7  88.99,37.73 180 top
R8  88.98,39.2 0 top
R9  79.51,76.34 0 top
R10  88.76,45.99 90 top
R11  87.25,45.98 270 top
R12  99.52,31.52 0 top
R13  69.73,37.79 0 top
R14  69.76,39.34 180 top
R15  43.37,23.85 90 top
R16  54.89,82.89 0 top
R17  57.87,81.39 180 top
R18  56.78,42.42 0 top
R19  30.79,23.77 90 top
R20  29.38,23.77 90 top
R21  27.97,23.77 90 top
R22  23.66,23.77 90 top
R23  22.23,23.78 90 top
R24  56.77,43.89 0 top
R27  16.91,64.16 0 top
R28  16.85,27.17 0 top
R29  16.92,46.5 0 top
R30  16.92,40.53 0 top
R31  16.92,44.49 180 top
R32  80.14,39.03 0 top
R33  80.22,27.95 180 top
R34  77.32,31.97 270 top
R35  77.3,35.02 90 top
R172  48.97,54.97 270 top
U1  85.74,31.92 270 top
U2  70.12,41.78 90 top
U3  81.44,69.17 270 top
U4  75.94,21.01 270 top
U5  20.68,82.66 0 top
U6  99.53,34.54 270 top
U$30  [LOGO-1]  23.38,51.04 0 top
U$42  [LOGO-MIN]  29.53,51.64 0 top

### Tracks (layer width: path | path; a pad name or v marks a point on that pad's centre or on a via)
3V3  (via drill 0.35)
  Top 0.254: v58.17,33.98 58.17,35.36 C24.1 | U4.16 v74.19,24.74 74.69,24.23 U4.15 | 71.58,32.82 71.58,32.85 | 78.75,71.99 78.74,71.99
  Top 0.5: Q8.1 81.02,37.79 81.02,38.92 R32.2 80.91,39.69 79.67,40.92 v78.65,40.92 | Q7.1 79.46,29.21 R33.2 79.28,27.95 v78.23,29 | L1.2 74.93,38.73 | C10.2 | 74.94,32.8 C11.2 | L2.1 53.93,54.93 C22.2 53.88,57.72 | 74.91,31.23 75.48,31.23 75.48,28.98 v75.63,28.98 | 20.48,46.56 20.48,57.74 20.48,61.36 R27.2 | 20.48,46.56 20.48,44.45 | 20.48,44.45 20.48,40.33 | 20.48,40.33 20.48,30.04 R28.2 | R30.2 20.29,40.53 20.48,40.33 | R31.1 20.44,44.49 20.48,44.45 | R29.2 17.75,46.56 20.48,46.56 | 37.58,57.74 37.6,57.72 37.63,57.69 C19.2 C18.2 C17.2 30.86,24.61 R19.2 R20.2 R21.2 26.94,24.54 | 26.94,24.54 R22.2 R23.2 | J1.4 v26.91,18.77 26.91,24.51 26.94,24.54 | U3.2 98.18,71.47 95.21,74.45 C12.2 C13.2 90.22,74.45 C14.2 89.22,74.43 86.78,71.99 78.74,71.99 58.54,71.99 | 58.54,71.99 53.6,71.99 48.81,67.19 48.81,65.69 | 58.54,71.99 58.64,72.08 R17.1 | 48.81,65.69 48.81,57.72 | 48.81,65.69 48.78,65.66 U5.11 U5.12 v41.08,70.66 U5.13 U5.14 | C24.1 51.58,42.41 51.96,42.79 v51.96,46.21 | R13.2 70.5,33.93 | v48.95,49.24 47.42,50.77 47.42,57.72 | R9.1 78.75,71.99 | 71.58,32.82 71.58,33.26 v72.12,33.8
  Top 1: 74.93,38.73 C9.2 C10.2 | C10.2 74.94,32.8 | C11.2 74.91,31.23 73.16,31.23 71.58,32.82 | 37.6,57.72 47.42,57.72 48.81,57.72 53.88,57.72 62.86,57.72 66.55,54.03 66.55,37.87 70.5,33.93 71.58,32.85 | 37.58,57.74 20.48,57.74
  Bottom 0.254: v74.19,24.74 74.19,25.46 72.67,26.97 64.98,26.97 58.17,33.79 v58.17,33.98 58.17,35.37 55.68,37.85 P69.P$1 | v72.12,33.8 72.12,34.87 P7.P$1 | v26.91,18.77 v26.9,18.78 P12.P$1
  Bottom 0.5: v78.65,40.92 78.23,40.5 v78.23,29 78.21,29.03 75.68,29.03 v75.63,28.98 | v51.96,46.21 51.96,46.23 v48.95,49.24 | v41.08,70.66 39.91,70.66 P27.P$1
  pour Top: 20.39,41.63 19.31,40.55 19.31,40.53 20.46,39.38 20.46,41.55 20.4,41.61
  pour Top: 20.49,48.35 20.42,48.18 19.71,46.57 20.42,45.48 20.49,44.98
  pour Top: 20.41,45.11 19.73,44.43 20.47,43.68 20.47,45.1 20.46,45.11
  pour Top: 45.79,57.84 47.46,56.17 49.03,57.74
  pour Top: 49.85,57.77 49.81,57.81 47.76,57.81
  pour Top: 48.73,66.41 48.75,65.88 48.75,66.39
  pour Top: 58.57,73.01 57.58,72.02 59.58,72.02 58.59,73.01
  pour Top: 20.49,58.69 20.5,56.74 20.5,58.68
  pour Top: 20.46,59.04 21.73,57.77 20.45,56.49 20.45,59.04
  pour Top: 36.3,57.72 37.68,56.35 39.04,57.71 39.03,57.72
  pour Top: 47.87,57.76 49.66,57.75 47.85,57.75
  pour Top: 48.93,67.51 47.97,66.55 48.92,65.6 48.93,65.47
  pour Top: 73.48,31.25 75.48,31.25 75.48,28.98
3V3_RX  (via drill 0.35)
  Top 0.254: Q8.2 79.29,38.95 R32.1 79.29,39.12 v79.29,40.1 | v93.94,52.6 94.37,52.17 U3.36
  Bottom 0.254: v93.94,52.6 93.94,52.57 87.62,46.25 87.62,34.8 87.01,34.19 85.7,34.19 85.31,34.58 85.31,37.64 82.83,40.12 79.32,40.12 79.32,40.13 v79.29,40.1
3V3_TX  (via drill 0.35)
  Top 0.254: v81.92,27.26 81.68,27.26 R33.1 80.99,29.09 Q7.2 | U3.37 95.64,51.97 v95.01,52.6
  Bottom 0.254: v95.01,52.6 95.01,52.58 88.21,45.78 88.21,34.78 87.16,33.73 85.64,33.73 85.22,33.31 85.22,29.33 83.15,27.26 v81.92,27.26
5V_RX
  Top 0.254: Q7.3 80.28,32.26 R6.1 77.35,32.76 R34.1
5V_TX
  Top 0.254: Q8.3 80.24,34.72 R5.1 77.33,34.23 R35.1
BAT  (via drill 0.35)
  Top 0.5: U6.3 98.53,36.31 v101.64,39.42 101.69,39.48 B1.1 | C5.2 C6.2 93.12,35.88 Q3.3 93.12,38.74 91.86,40.01 D3.A
  Top 0.6: B1.1 100.62,42.98 97.49,39.85 97.49,37.49 95.71,35.71 C5.2
  Bottom 0.254: v101.64,39.42 99.82,39.42 P5.P$1
BOOT  (via drill 0.35)
  Top 0.254: v70.91,55.74 70.91,54.13 73.87,51.17 U3.27 79.97,51.14 79.97,50.19 80.5,49.66 v81.43,49.66 | v69.83,72.82 66.55,76.1 66.55,79.97 K1.2 | v84.02,47.16 84.02,47.05 88.38,42.7 Q2.3
  Bottom 0.254: v70.91,55.74 70.91,71.74 v69.84,72.82 v69.83,72.82 | v84.02,47.16 81.52,49.66 v81.43,49.66
D+
  Top 0.254: J2.B6 97.57,23.77 | 97.57,23.77 96.81,23.77 94.93,23.77 93.38,23.77 R3.1 | 97.57,23.77 97.57,23.16 97.97,22.76 J2.A6
D-
  Top 0.254: R2.1 93.27,22.26 J2.B7 99.98,22.26 100.17,22.45 100.17,23 99.91,23.26 J2.A7
DTR  (via drill 0.35)
  Top 0.254: v89.56,32.55 U1.13 | R7.1 90.3,37.73 90.71,37.32 v90.75,37.32 90.7,37.37 90.7,39.88 Q2.2
  Bottom 0.254: v89.56,32.55 90.7,33.69 90.7,37.28 v90.75,37.32
EN_RESET  (via drill 0.35)
  Top 0.254: v93.89,56.27 96.9,59.28 U3.3 96.91,70.84 95.54,72.21 92,72.21 v91.48,72.73 | v88.72,75.44 86.36,77.8 C2.2 | Q1.3 86.28,40.18 86.8,40.69 v86.8,40.93 | C2.2 80.27,79.99 K2.2 | R9.2 80.28,77.79 C2.2
  Bottom 0.254: v91.48,72.73 v91.48,72.74 88.78,75.44 v88.72,75.44 | v93.89,56.27 93.82,56.2 93.82,56.22 86.8,49.2 v86.8,40.93
GDR  (via drill 0.35)
  Top 0.254: v59.22,39.53 57.55,41.21 R18.2 56.81,43.16 56.81,48.7 55.84,49.66 55.84,50.49 Q4.1 | v60.94,33.99 v60.95,33.99 60.95,39.55 v60.93,39.57 | v81.18,24.9 v81.19,24.89 U4.2
  Bottom 0.254: v60.93,39.57 59.25,39.57 | 59.25,39.57 v59.22,39.53 | v81.18,24.9 80.29,25.8 75.64,25.8 73.18,28.26 66.57,28.26 60.94,33.89 v60.94,33.99 | P66.P$1 59.2,39.62 59.25,39.57
GND  (via drill 0.35, 3.2 pad 5)
  Top 0.254: J2.B1 J2.A12 | v96.53,19.81 96.56,19.84 98.79,19.84 J2.A1 J2.B12 | v101.04,45.19 101.4,44.84 101.69,44.49 B1.2 | Q10.2 v39.59,27
  Top 0.5: U5.9 v41.14,75.66 | Q9.2 v50.44,51.19 v50.43,51.18
  Bottom 0.254: v96.53,19.81 95.72,19 P1.P$1 | v101.04,45.19 99.82,45.19 P6.P$1 | P13.P$1 39.59,28.53 v39.59,27
  Bottom 0.5: P44.P$1 v50.43,51.18 | P35.P$1 41.12,75.68 v41.14,75.66
  other vias: 4,83 103,83 83.49,43.49 23.49,43.49 4,4 103,4 48.81,51.2 46.22,48.37 48.46,31.66 47.17,27.13 97.7,29.91 95.31,17.2 97.08,15.97 95.9,29.76 60.13,20.42 64.66,21.24 53.96,66.64 56.69,69.76 62.8,70.26 66.1,70.39 67.99,66.27 61.07,42.52 77.2,29.91 55.41,52.49 56.7,52.23 59.97,56.65 54.52,49 76.53,37.28 72.53,37.82 72.69,40.73 73.39,41.56 78.47,43.58 79.12,42.29 15.97,80.24 13.83,77.16 17.18,60.16 20.62,63.1 17.27,53.91 22.06,55.48 22.19,60.31 21.43,46.4 21.52,36.12 14.48,22.25 9.59,17.59 12.55,14.85 18.16,17.77 17.35,12.34 17.39,7.31 39.9,18.53 45.64,8.66 51.87,8.16 41.56,32.23 44.02,35.98 38.58,52.3 90.34,27.27 60.13,10.94 68.15,10.87 78.97,10.92 87.59,16.81 87.6,10.96 91.32,18.59 93.11,11.08 102.8,23.58 89.56,28.19 99.24,48.94 43.84,56.39 42.81,59.05 33.46,58.82 22.59,65.02 47.64,84.06 61.94,83.89 78.13,83.67 92.23,80.48 95.58,77.77 29.79,62.27 87,65.35 87.37,62.46 87.46,59.22 88.19,56.81 90.3,57.36 90.68,65.62 65.35,30.85 67.74,30.86 66.88,29.16 69.09,29.14 52.98,21.33 64.85,23.72 66.74,23.74 66.43,21.19 52.31,27.64 85.89,46.29 89.97,17.15 55.92,24.12 48.8,52.67 51.58,49.78 74.05,55.63 75.67,55.61 67.7,50.97 67.66,48.19 67.7,43.32 52.9,43.98 52.92,42.3 99.61,32.97 97.55,36.21 97.12,35.11 97.01,33.84 97.56,32.17 98.17,34.57 99.48,34.46 100.81,34.49 100.32,36.9 101.58,36.26 101.97,34.6 101.83,33.41
  pour Top (rank 2): -6.75,88.42 -6.75,-2.41 112,-2.41 112,45.89 99.95,45.89 99.95,77.69 109.13,77.69 109.13,88.4 -6.73,88.4
  pour Bottom: -6.86,88.57 -6.86,-2.35 111.56,-2.35 111.56,45.95 99.96,45.95 99.96,77.69 99.95,77.69 109.21,77.69 109.21,88.58 -6.87,88.58
IO1_EXIT  (via drill 0.35)
  Top 0.254: K4.2 6.42,27.18 v7.89,27.18 16.08,27.18 R28.1 | U3.39 v98.19,52.53
  Bottom 0.254: v7.89,27.18 7.89,21.44 15.61,13.72 90.33,13.72 94.8,18.19 94.8,49.24 98.1,52.53 v98.19,52.53
IO2_MENU  (via drill 0.35)
  Top 0.254: K3.2 7.46,67.05 v10.4,64.11 16.1,64.11 R27.1 | v96.93,52.59 96.91,52.61 U3.38
  Bottom 0.254: v10.4,64.11 10.4,21.19 17.33,14.26 90.18,14.26 93.93,18.01 93.93,49.59 v96.93,52.59
IO3  (via drill 0.35)
  Top 0.254: U3.15 v76.81,67.17 v76.8,67.16 | v38.18,77.86 v22.74,77.86 22.08,77.2 U5.1
  Bottom 0.254: v76.8,67.16 76.8,72.66 71.6,77.86 v38.18,77.86 | v22.74,77.86 22.07,77.19 P28.P$1
IO4_DOWN  (via drill 0.35)
  Top 0.254: R30.1 v11.46,40.53 9.22,40.53 K5.1 | v95.66,70.83 95.66,69.19 U3.4
  Bottom 0.254: v95.66,70.83 95.66,74.2 86.99,82.87 21.99,82.87 11.46,72.34 v11.46,40.53
IO5_CONF  (via drill 0.35)
  Top 0.254: R31.2 v12.42,44.49 9.22,44.49 K5.4 | U3.5 94.37,70.89 v94.36,70.86
  Bottom 0.254: v94.36,70.86 94.36,74.26 86.2,82.42 23.08,82.42 12.42,71.76 v12.42,44.49
IO6_UP  (via drill 0.35)
  Top 0.254: K5.2 9.21,46.5 v13.64,46.5 R29.1 | v93.15,70.79 93.15,69.22 U3.6
  Bottom 0.254: v93.15,70.79 93.15,74.34 85.53,81.96 24.46,81.96 13.64,71.14 v13.64,46.5
IO7_LCD_3.3_CTL  (via drill 0.35)
  Top 0.254: U3.7 91.83,68.38 91.48,68.03 67.83,68.03 64.36,64.56 v64.36,61.91 | v52.47,56.66 51.55,55.74 R172.1
  Bottom 0.254: v64.36,61.91 64.1,61.65 57.46,61.65 v52.47,56.66
IO8  (via drill 0.35)
  Top 0.254: v85.5,70.69 85.5,69.19 U3.12 | v33.86,79.09 22.77,79.09 20.5,76.82 20.5,72.24 v20.69,72.05 U5.20
  Bottom 0.254: v85.5,70.69 85.5,72.17 78.19,79.48 34.23,79.48 33.86,79.11 v33.86,79.09 | P20.P$1 20.72,72.05 v20.69,72.05
IO9  (via drill 0.35)
  Top 0.254: v46.51,64.63 43.23,61.35 28.12,61.35 25.47,64 v25.47,73.94 25.47,74.81 U5.2 | U3.17 v67.04,64.62
  Bottom 0.254: v67.04,64.62 67.02,64.64 47.43,64.64 47.42,64.63 v46.51,64.63 | P29.P$1 25.47,74.82 v25.47,73.94
IO10_SPI_CS  (via drill 0.35)
  Top 0.254: v55.64,60.99 55.83,61.18 68.89,61.18 71.08,63.37 78.42,63.37 U3.18 | R20.1 29.4,22.99 v29.4,21.55 v29.4,21.54 29.11,21.25 J1.2
  Bottom 0.254: v29.4,21.55 29.4,22.79 | 29.4,22.79 29.4,34.72 55.64,60.96 v55.64,60.99 | P8.P$1 29.43,22.76 29.4,22.79
IO11_SPI_MOSI  (via drill 0.35)
  Top 0.254: v86.16,62.08 U3.19 | U4.14 75.19,24.69 65.81,34.08 v65.73,34.08
  Bottom 0.254: v86.16,62.08 86.16,55.37 65.73,34.94 v65.73,34.08 67.46,32.35 P55.P$1
IO12_SPI_CLK  (via drill 0.35)
  Top 0.254: U4.13 75.69,23.65 75.7,23.66 75.7,25.06 65.68,35.08 v65.05,35.08 | U3.20 85.31,60.81 v85.35,60.77
  Bottom 0.254: v65.05,35.08 65.1,35.08 85.4,55.38 85.4,60.72 v85.35,60.77 | v65.05,35.08 | v65.05,35.08 P54.P$1
IO13_SPI_MISO  (via drill 0.35)
  Top 0.254: J1.7 v23.61,21.54 23.61,22.96 R22.1 | v50.24,60.08 50.46,60.08 50.46,60.07 80.15,60.07 80.68,59.54 U3.21
  Bottom 0.254: 23.62,22.8 23.62,33.45 v50.24,60.08 | 23.62,22.8 23.62,21.74 23.61,21.73 v23.61,21.54 | P11.P$1 23.6,22.78 23.62,22.8
IO14  (via drill 0.35)
  Top 0.254: v70.21,58.23 70.25,58.27 U3.22 | v47.7,63.98 46.94,63.98 43.76,60.8 27.57,60.8 24.62,63.75 v24.62,68.89 U5.19
  Bottom 0.254: v70.21,58.23 70.14,58.3 70.14,59.65 65.82,63.98 v47.7,63.98 | v24.62,68.89 v24.61,68.9 P21.P$1
IO15  (via drill 0.35)
  Top 0.254: U3.8 v90.56,70.75 v90.57,70.76 | U5.3 27.16,76.45 27.89,77.18 v27.92,77.18
  Bottom 0.254: v90.57,70.76 90.57,72.59 81.69,81.47 32.21,81.47 v27.92,77.18 27.15,76.41 P30.P$1
IO16  (via drill 0.35)
  Top 0.254: v89.26,70.72 89.26,69.18 U3.9 | U5.18 27.16,72.39 v27.19,72.42
  Bottom 0.254: v89.26,70.72 89.26,72.44 80.8,80.91 32.61,80.91 28.15,76.45 28.15,73.38 v27.19,72.42 27.17,72.4 P22.P$1
IO17  (via drill 0.35)
  Top 0.254: v88.03,70.74 88.02,70.72 U3.10 | v30.04,77.2 29.7,76.86 U5.4
  Bottom 0.254: v88.03,70.74 88.03,72.27 79.96,80.35 33.19,80.35 v30.04,77.2 29.71,76.87 P31.P$1
IO18  (via drill 0.35)
  Top 0.254: U3.11 86.78,69.2 v86.78,70.77 | v29.72,72.42 29.72,70.68 U5.17
  Bottom 0.254: v86.78,70.77 86.78,72.13 78.98,79.93 33.77,79.93 31.35,77.51 31.35,74.05 v29.72,72.42 29.69,72.39 P23.P$1
IO19  (via drill 0.35)
  Top 0.254: v84.22,70.69 U3.13 | v33.34,76.76 | U5.5 v33.34,76.76
  Bottom 0.254: v84.22,70.69 84.22,71.75 77.04,78.93 35.6,78.93 33.43,76.76 v33.34,76.76 32.28,75.7 P32.P$1
IO20  (via drill 0.35)
  Top 0.254: v82.93,70.7 U3.14 | v32.22,72.46 32.24,72.44 U5.16
  Bottom 0.254: v82.93,70.7 75.11,78.52 36.17,78.52 33.33,75.68 33.33,73.56 v32.22,72.46 | v32.22,72.46 | P24.P$1 32.22,70.64 v32.22,72.46
IO21  (via drill 0.35)
  Top 0.254: v42.89,63.28 36.57,63.28 35.78,64.07 v35.78,73.32 35.78,74.66 U5.6 | v69.49,57.16 78.28,57.16 U3.23
  Bottom 0.254: v42.89,63.28 65.61,63.28 69.49,59.39 v69.49,57.16 | P33.P$1 35.78,74.59 v35.78,73.32
IO38  (via drill 0.35)
  Top 0.254: v68.84,56.4 68.84,55.17 75.08,48.93 82.05,48.93 82.95,49.83 87.43,49.83 88.02,50.42 U3.31 | v41.79,62.61 36.03,62.61 34.72,63.92 v34.72,68.7 34.72,70.6 U5.15
  Bottom 0.254: v68.84,56.4 68.75,56.49 68.75,59.48 65.62,62.61 v41.79,62.61 | P25.P$1 34.75,68.73 v34.72,68.7
IO39_SPI_CLK  (via drill 0.35)
  Top 0.254: U3.32 89.29,50.54 88.08,49.33 83.02,49.33 82.22,48.53 74.92,48.53 63.84,59.6 51.11,59.6 v50.92,59.41 | v25.79,21.43 25.79,14.64 J1.5
  Bottom 0.254: v50.92,59.41 25.79,34.28 v25.79,21.43 24.59,20.23 P10.P$1
IO40_SPI_MOSI  (via drill 0.35)
  Top 0.254: U3.33 90.56,50.74 88.68,48.85 83.12,48.85 82.39,48.12 74.75,48.12 63.95,58.91 v51.7,58.91 v51.69,58.92 | v28,21.19 v28.01,21.18 | v28.01,21.18 J1.3 | R21.1 28.01,22.97 v28.01,21.18
  Bottom 0.254: v51.69,58.92 28,35.23 v28,21.19 28.98,20.21 P9.P$1
IO41_LED  (via drill 0.35)
  Top 0.254: v71.65,56.5 71.65,54.11 73.36,52.4 91.42,52.4 91.83,51.99 U3.34 | R16.1 54.16,82.86 54.06,82.76 v54.06,76.87
  Bottom 0.254: v71.65,56.5 71.65,56.53 71.52,56.66 71.52,72.08 66.73,76.87 v54.06,76.87
IO42_TF_3.3_CTL  (via drill 0.35)
  Top 0.254: v43.47,21.43 43.47,23.02 R15.1 | v95.98,52.61 95.28,53.31 93.69,53.31 93.1,52.72 U3.35
  Bottom 0.254: v43.47,21.43 49.54,15.36 89.95,15.36 93.53,18.94 93.53,50.13 95.98,52.59 v95.98,52.61
IO45_CS  (via drill 0.35)
  Top 0.254: U4.12 76.18,25.15 65.35,35.99 v64.88,35.99 | v82.86,53.77 82.26,53.17 U3.26
  Bottom 0.254: v82.86,53.77 65.08,35.99 v64.88,35.99 62.85,33.96 P53.P$1
IO46_D/C  (via drill 0.35)
  Top 0.254: U4.11 76.69,25.34 65.01,37.02 v64.71,37.02 | U3.16 83.86,65.89 v84.06,66.09
  Bottom 0.254: v84.06,66.09 84.15,66 84.15,56.02 65.15,37.02 v64.71,37.02 64.69,37.02 63.54,35.86 P52.P$1
IO47_RES  (via drill 0.35)
  Top 0.254: v64.83,38.16 64.83,37.85 77.19,25.49 U4.10 | v82.92,55.76 82.89,55.73 U3.24
  Bottom 0.254: v82.92,55.76 82.78,55.9 64.94,38.06 v64.83,38.16 v64.82,38.17 P51.P$1
IO48_BUSY  (via drill 0.35)
  Top 0.254: v79.79,54.44 79.77,54.46 U3.25 | U4.9 77.7,25.58 65.5,37.77 v65.5,39.61
  Bottom 0.254: v79.79,54.44 79.33,53.98 79.31,53.98 65.5,40.17 v65.5,39.61 64.93,40.18 P50.P$1
LCD_GND  (via drill 0.35)
  Top 0.254: U4.17 73.69,22.7 | U4.6 79.19,22.75 79.08,22.64 | 78.64,22.64 78.69,22.69 U4.7 78.69,22.74 78.65,22.7 78.19,22.7 U4.8 78.19,22.7 78.13,22.64 | C22.1 53.94,53.3
  Top 0.5: C22.1 52.56,53.36 Q9.3 52.47,48.63 52.47,48.62 | D5.C 62.46,45.35 C20.1 62.61,45.17 v62.61,43.94 | R18.1 56.01,42.43 R24.1 54.29,43.89 | 54.29,43.89 54.36,43.82 v54.36,46.74 52.47,48.62 | 54.29,43.89 C23.2 | C24.2 C25.2 C26.2 | C26.2 C27.2 C28.2 | v59.29,43.93 59.26,43.97 C29.1 v59.26,46.72 | C26.2 48.29,46.92 49.99,48.62 52.47,48.62 | 73.69,22.7 73.69,22.34 | 73.69,22.34 73.69,19.71 71.47,17.49 64.88,17.49 62.59,19.78 v62.59,41.28 | 73.69,22.34 v75.02,22.34 77.84,22.34 78.13,22.64 78.64,22.64 79.08,22.64 | 53.94,53.3 v53.94,51.52
  Bottom 0.254: P43.P$1 53.94,50.38
  Bottom 0.5: v59.29,43.93 v59.3,43.94 v62.61,43.94 62.59,43.92 v62.59,41.28 | v59.26,46.72 54.37,46.72 v54.36,46.74 | 53.94,50.38 v53.94,51.52 | P68.P$1 v75.02,22.34
N$1
  Top 0.254: Q1.1 85.59,37.29 87.79,37.29 R7.2
N$2
  Top 0.254: U1.2 82.15,35.09 R5.2
N$3
  Top 0.254: U1.3 82.37,33.82 R6.2
N$4
  Top 0.254: R8.2 88.28,40.67 Q2.1
N$5
  Top 0.254: J2.A5 94.18,21.76 R1.2
N$6
  Top 0.254: R11.1 R10.2 89.48,47.47 91.9,47.47 94.13,45.24 94.13,38.78 Q3.1
N$7
  Top 0.254: R172.2 50.43,54.21 Q9.1
N$8
  Top 0.254: R15.2 43.25,24.62 42.74,25.12 41.52,25.12 Q10.1
N$9
  Top 0.254: R13.1 68.97,39.31 R14.2 69,40.76 U2.5
N$10
  Top 0.254: J1.1 30.21,21.46 30.79,22.04 R19.1
N$11
  Top 0.7: U2.3 74.61,42.73 L1.1
  pour Top: 71.23,42.78 72.4,43.95 75.07,43.95 75.07,42.49 75.01,42.43 71.58,42.43
N$12
  Top 0.254: J2.B5 93.52,24.76 R4.1
N$13
  Top 0.254: C15.1 83.27,37.93 84.65,36.56 84.65,33.03 84.17,32.55 U1.4
N$16
  Top 0.254: U6.5 100.53,31.76 R12.2
N$20
  Top 0.254: J1.8 22.51,22.74 R23.1
N$25
  Top 0.254: R17.2 57.11,82.85 D1.+ R16.2
N$55
  Top 0.5: C21.1 63.36,53.37 63.36,53.36 | 63.36,53.36 62.46,52.46 D5.A | D4.C 64.27,52.45 63.36,53.36
N$56
  Top 0.8: 60.7,55.26 58.91,55.26 L2.2 Q4.3 | D6.A 60.7,55.26 | C21.2 60.7,55.26
  pour Top: 58.27,55.95 60.87,55.95 60.87,52.89 60.76,52.78 58.27,52.78
PREVGH  (via drill 0.35)
  Top 0.254: D6.C 60.7,45.28 C29.2 60.79,44.56 63.29,42.06 63.29,20.13 65.04,18.39 70.72,18.39 71.69,19.36 71.69,21.98 | 71.69,21.98 U4.21 | 71.69,21.98 72.54,21.98 v72.57,21.95
  Bottom 0.254: v72.57,21.95 72.57,20.31 P56.P$1
PREVGL  (via drill 0.35)
  Top 0.254: D4.A 64.16,47.28 C20.2 64.16,42.62 63.7,42.16 63.7,20.29 65.2,18.79 69.95,18.79 70.69,19.53 v70.69,21.8 U4.23
  Bottom 0.254: P57.P$1 v70.69,21.8
RESE  (via drill 0.35)
  Top 0.254: Q4.2 57.54,49.17 R24.2 58.13,43.89 59.98,42.05 59.98,34.02 v60.01,34.02 | v80.2,24.92 80.69,24.43 U4.3
  Bottom 0.254: v80.2,24.92 v80.2,24.93 79.74,25.39 75.47,25.39 73.01,27.85 66.08,27.85 60.01,33.92 v60.01,34.02 60.01,37.88 P67.P$1
RTS  (via drill 0.35)
  Top 0.254: U1.14 86.58,33.82 86.02,34.38 v86.02,34.86 | Q1.2 86.64,39.26 v86.7,39.31 88.11,39.31 R8.1
  Bottom 0.254: v86.7,39.31 86.02,38.64 v86.02,34.86
TF_GND  (via drill 0.35)
  Top 0.254: Q10.3 v40.55,21.9
  Top 0.5: J1.6 24.71,13.5 26.14,12.07 30.16,12.07 34.83,16.74 C17.1
  Top 0.8: Q10.3 40.52,23.08 C19.1 C18.1 C17.1
  Bottom 0.254: v40.55,21.9 P45.P$1
USB_D+  (via drill 0.35)
  Top 0.254: R3.2 91.7,23.62 89.1,23.62 | 89.1,23.62 88.71,23.62 85.8,26.53 85.8,29.02 83.54,31.28 U1.5 | 89.1,23.62 89.06,23.66 v89.06,24.27
  Bottom 0.254: v89.06,24.27 P4.P$1
USB_D-  (via drill 0.35)
  Top 0.254: R2.2 89.04,22.22 | 89.04,22.22 88.63,22.22 85.03,25.82 85.03,28.49 83.51,30.01 U1.6 | 89.04,22.22 v89.04,21.52 v89.03,21.51
  Bottom 0.254: v89.03,21.51 P3.P$1
VBUS  (via drill 0.35)
  Top 0.254: J2.B9 98.97,20.59 J2.A4 | 95.62,25.41 95.69,25.48 v95.69,26.95 | 98.97,25.49 J2.A9 98.82,25.41 | 98.97,25.49 98.9,25.42 | J2.B4 98.97,25.49
  Top 0.5: v77.61,28.16 77.61,28.21 76.21,29.61 76.21,31.21 | 93.5,26.42 94.51,25.41 95.62,25.41 98.82,25.41 | U1.16 90.02,36.36 C1.1 90.47,36.21 v91.82,34.85 | v91.79,32.96 91.84,33.01 98.27,33.01 U6.4 | R35.2 76.41,35.79 76.21,35.59 76.21,31.21 | R34.2 76.21,31.21 | 98.9,25.42 99.97,25.42 100.94,24.45 100.94,21.63 99.9,20.59 98.97,20.59
  Top 0.6: C4.2 91.38,30.29 v91.38,26.46
  Top 0.7: C3.2 91.35,31.9 C4.2 | 93.5,26.42 91.42,26.42 v91.38,26.46
  Top 0.8: v90.24,42.79 90.24,44.72 D2.1 88.8,45.26 R10.1 | v91.79,32.96 91.79,32.34 C3.2
  Bottom 0.254: v95.69,26.95 P2.P$1
  Bottom 0.5: v91.38,26.46 91.38,26.41 79.35,26.41 v77.61,28.16
  Bottom 0.8: v91.79,32.96 91.79,34.82 v91.82,34.85 91.82,41.21 v90.24,42.79
VCOM  (via drill 0.35)
  Top 0.254: v70.17,24.83 70.17,23.57 U4.24 | C28.1 45.5,42.41 54.03,33.87 v54.49,33.87
  Bottom 0.254: v70.17,24.83 v70.16,24.83 69.65,25.35 63.02,25.35 v54.49,33.87 52.44,33.87 P73.P$1
VDD  (via drill 0.35)
  Top 0.254: v73.18,24.74 U4.18 | C25.1 49.7,41.52 v57.25,33.98
  Bottom 0.254: v73.18,24.74 v73.18,24.73 73.18,25.47 72.09,26.57 64.65,26.57 v57.25,33.97 v57.25,33.98 53.37,37.85 P70.P$1
VDHR  (via drill 0.35)
  Top 0.254: C23.1 54.58,42.41 59.08,37.9 v59.08,33.99 | v79,24.74 79.46,24.74 79.69,24.5 U4.5
  Bottom 0.254: v79,24.74 v79,24.73 75.55,24.73 72.84,27.44 65.63,27.44 v59.08,33.99 59.08,36.25 P58.P$1
VIN
  Top 0.6: D2.2 92.77,48.27 83.89,48.27 82.87,47.25 70.19,47.25 C8.2 68.86,44.21 C7.2 68.9,42.76 U2.4 68.92,42.34 70.43,40.83 U2.1
  Top 0.8: D2.2 95.91,45.14 D3.C 95.52,41.29 Q3.2
VSH  (via drill 0.35)
  Top 0.254: v72.2,24.83 U4.20 | v56.32,33.98 48.29,42 C26.1
  Bottom 0.254: v72.2,24.83 72.2,25.45 71.5,26.16 64.14,26.16 v56.32,33.98 | v56.32,33.98 | v56.32,33.98 53.61,36.68 50.58,36.68 P71.P$1
VSL  (via drill 0.35)
  Top 0.254: U4.22 v71.19,24.8 | C27.1 47.44,41.85 47.45,41.85 55.33,33.97 v55.4,33.97
  Bottom 0.254: v71.19,24.8 v71.18,24.8 71.18,25.37 70.8,25.76 63.61,25.76 v55.4,33.97 54.81,34.55 P72.P$1

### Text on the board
tPlace: H2 | H1 | IO3 | IO9 | IO15 | IO17 | IO19 | IO21 | GND | GND | GND | GND | IO2 | IO8 | IO14 | IO16 | IO18 | IO20 | IO38 | 3V3 | 3V3 | 3V3 | 3V3 | IO7 | ESP32 Display-4.2(E) inch | SKU:DIE07300S | V1.0 | - | H5 | H6 | + | IO6 / IO5 / IO4 | IO1 | IO42 | IO10 => SPI_CS / IO40 => SPI_MOSI / IO39 => SPI_CLK / IO13 => SPI_MISO | E-paper | IO48 => LCD_BUSY / IO47 => LCD_RES / IO46 => LCD_D/C / IO45 => LCD_SPI_CS / IO12 => LCD_SPI_CLK / IO11 => LCD_SPI_MOSI | H3 | H4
